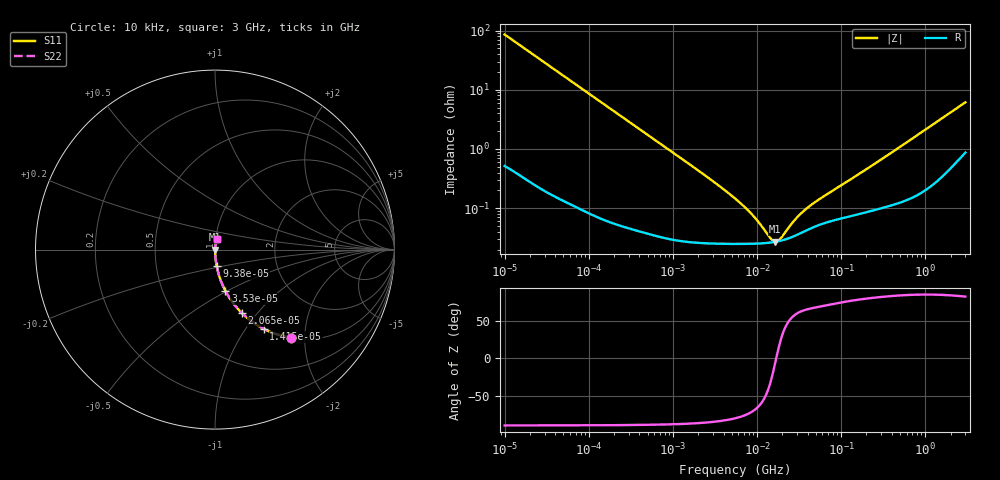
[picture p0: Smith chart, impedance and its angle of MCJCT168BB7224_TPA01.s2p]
! MCJCT168BB7224_TPA01  S-PARAMETER MODEL  ( Standard Model )
! Model Generated by TAIYO YUDEN Corporation (http://www.ty-top.com)
! Version 1.0
! TAIYO YUDEN Control No. 220601
! Copyright(c) 2015 TAIYO YUDEN CO.,LTD. All Rights Reserved.
! Product Description (link to TY-COMPAS)
! https://ds.yuden.co.jp/TYCOMPAS/or/detail?pn=MCJCT168BB7224KTPA01&u=M
! Products Name : Multilayer Ceramic Capacitors
! Characteristics :
!  Capacitance : 0.22 [uF] , Rated Voltage : 25 [V] , TCC : X7R
!  Case Size : 1.6 x 0.8 / 0.063 x 0.031 [mm/inch] , Thickness : 0.8 / 0.031 [mm/inch]
!  (Conditions: Temperature = 25 [degC] , DC Bias Voltage = 0 [V])
! External Node Assignments :
!  1  o---| |---o  2
! GND o---------o GND
! Frequency Range : 10kHz  -  3GHz  [ 401 STEP ]
# MHZ S RI R 50
! Freq[MHz].  S11 Real  S11 Imag  S21 Real  S21 Imag  S12 Real  S12 Imag  S22 Real  S22 Imag
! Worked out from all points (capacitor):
!   401 points, 10 kHz to 3 GHz, reference 50 ohm
!   read as one part in series: C = 185 nF near 10.65 kHz
!   lowest |Z| = 27.1 mohm at 16.51 MHz (marker M1)
!   series resonance near 16.95 MHz, so ESL is about 480 pH
!   S11 on the Smith chart (normalised r, x): 10 kHz: 1.01, -1.72; 14.15 kHz: 1.01, -1.22; 20.65 kHz: 1.01, -0.83; 35.3 kHz: 1.00, -0.49; 93.8 kHz: 1.00, -0.18; 3 GHz: 1.02, +0.12
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0.01  0.4248 -0.4913  0.5752 0.4913  0.5752 0.4913  0.4248 -0.4913
0.014146  0.2711 -0.4414  0.7289 0.4414  0.7289 0.4414  0.2711 -0.4414
0.020651  0.1497 -0.3536  0.8503 0.3536  0.8503 0.3536  0.1497 -0.3536
0.035295  0.0578 -0.2299  0.9422 0.2299  0.9422 0.2299  0.0578 -0.2299
0.053176  0.0269 -0.1579  0.9731 0.1579  0.9731 0.1579  0.0269 -0.1579
0.082683  0.0117 -0.1034  0.9883 0.1034  0.9883 0.1034  0.0117 -0.1034
0.093797  0.00929 -0.0914  0.9907 0.0914  0.9907 0.0914  0.00929 -0.0914
0.219733  0.00208 -0.0395  0.9979 0.0395  0.9979 0.0395  0.00208 -0.0395
0.683653  0.000492 -0.0128  0.9995 0.0128  0.9995 0.0128  0.000492 -0.0128
2.652321  0.000264 -0.00323  0.9997 0.00323  0.9997 0.00323  0.000264 -0.00323
5.477226  0.000251 -0.00144  0.9997 0.00144  0.9997 0.00144  0.000251 -0.00144
8.516475  0.000251 -0.000774  0.9997 0.000774  0.9997 0.000774  0.000251 -0.000774
10.61963  0.000254 -0.000505  0.9997 0.000505  0.9997 0.000505  0.000254 -0.000505
14.55585  0.000263 -0.000159  0.9997 0.000159  0.9997 0.000159  0.000263 -0.000159
16.51234  0.00027 -2.7e-05  0.9997 2.7e-05  0.9997 2.7e-05  0.00027 -2.7e-05
18.73182  0.00028 0.000104  0.9997 -0.000104  0.9997 -0.000104  0.00028 0.000104
29.12589  0.000349 0.000572  0.9997 -0.000572  0.9997 -0.000572  0.000349 0.000572
35.19136  0.000396 0.00078  0.9996 -0.00078  0.9996 -0.00078  0.000396 0.00078
45.28751  0.000467 0.00107  0.9995 -0.00107  0.9995 -0.00107  0.000467 0.00107
374.4521  0.00115 0.00811  0.9988 -0.00811  0.9988 -0.00811  0.00115 0.00811
1202.347  0.00305 0.0252  0.997 -0.0252  0.997 -0.0252  0.00305 0.0252
3000  0.0122 0.0594  0.9878 -0.0594  0.9878 -0.0594  0.0122 0.0594
